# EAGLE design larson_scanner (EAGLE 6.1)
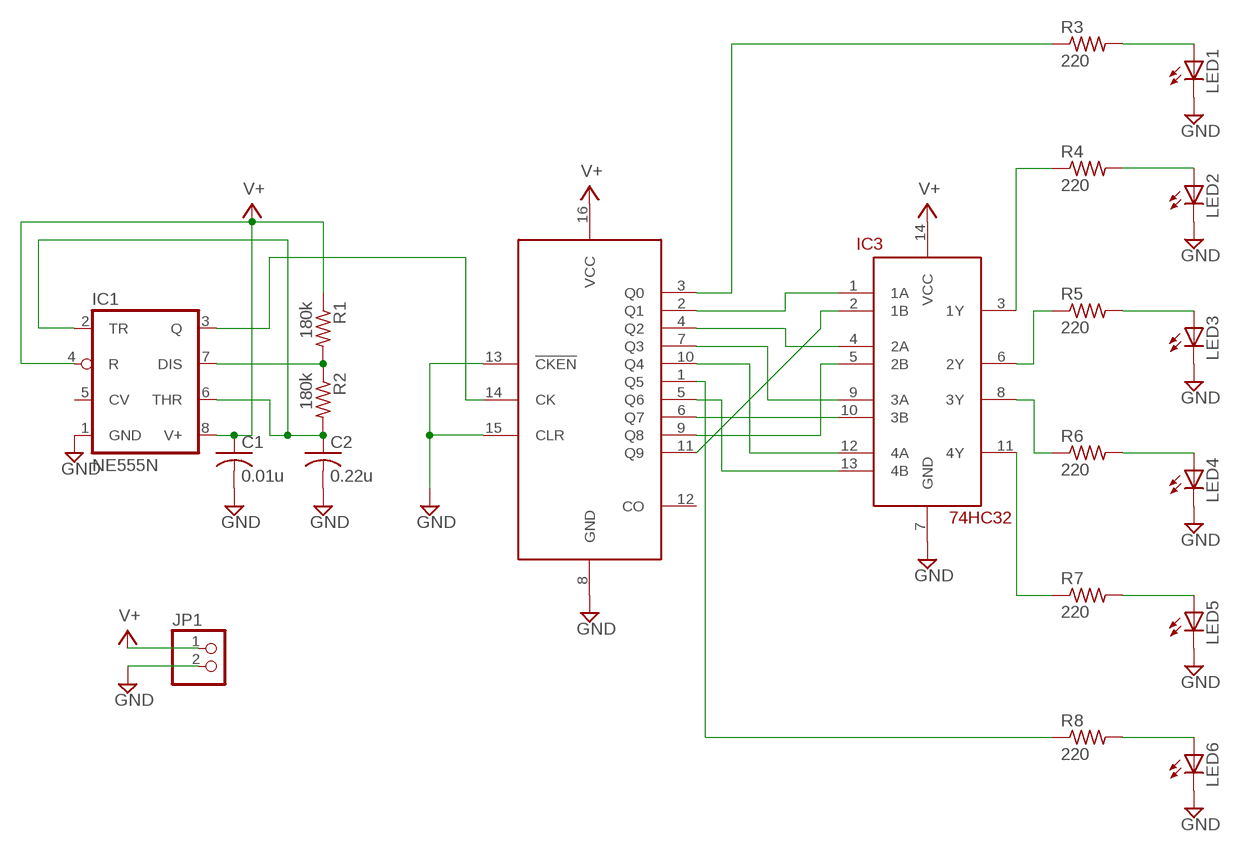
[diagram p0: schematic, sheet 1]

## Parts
C1  0.01u  C-US025-025X050  [C025-025X050]
C2  0.22u  C-US025-025X050  [C025-025X050]
IC1  NE555N  [DIL08]
IC2  74HC4017  [DIP16]
IC3  74HC32  [DIP14]
JP1  PINHD-1X2  [1X02]
LED1  LED5MM  [LED5MM]
LED2  LED5MM  [LED5MM]
LED3  LED5MM  [LED5MM]
LED4  LED5MM  [LED5MM]
LED5  LED5MM  [LED5MM]
LED6  LED5MM  [LED5MM]
R1  180k  R-US_0204/7  [0204/7]
R2  180k  R-US_0204/7  [0204/7]
R3  220  R-US_0204/7  [0204/7]
R4  220  R-US_0204/7  [0204/7]
R5  220  R-US_0204/7  [0204/7]
R6  220  R-US_0204/7  [0204/7]
R7  220  R-US_0204/7  [0204/7]
R8  220  R-US_0204/7  [0204/7]

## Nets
GND: C1.2 C2.2 IC1.1(GND) IC2.8(GND) IC2.13(!CKEN) IC2.15(CLR) IC3.7(GND) JP1.2 LED1.K(C) LED2.K(C) LED3.K(C) LED4.K(C) LED5.K(C) LED6.K(C)
N$1: LED4.A R6.2
N$2: LED3.A R5.2
N$3: LED2.A R4.2
N$4: LED1.A R3.2
N$5: LED5.A R7.2
N$6: LED6.A R8.2
N$7: IC2.1(Q5) R8.1
N$8: IC3.3(1Y) R4.1
N$9: IC3.6(2Y) R5.1
N$10: IC3.8(3Y) R6.1
N$11: IC2.3(Q0) R3.1
N$12: IC3.11(4Y) R7.1
N$13: IC2.2(Q1) IC3.1(1A)
N$14: IC2.4(Q2) IC3.4(2A)
N$15: IC2.7(Q3) IC3.9(3A)
N$16: IC2.10(Q4) IC3.12(4A)
N$17: IC2.5(Q6) IC3.13(4B)
N$18: IC2.6(Q7) IC3.10(3B)
N$19: IC2.9(Q8) IC3.5(2B)
N$20: IC2.11(Q9) IC3.2(1B)
N$21: IC1.7(DIS) R1.2 R2.1
N$22: C2.1 IC1.2(TR) IC1.6(THR) R2.2
N$23: IC1.3(Q) IC2.14(CK)
V+: C1.1 IC1.4(R) IC1.8(V+) IC2.16(VCC) IC3.14(VCC) JP1.1 R1.1
Unconnected: IC1.5(CV) IC2.12(CO)

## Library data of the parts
C1 C2 = rcl:C-US: CAPACITOR, American symbol
IC1 = linear:*555: TIMER
IC2 = jcm:74HC4017: Decimal counter with carry
IC3 = jcm:74HC32
JP1 = pinhead:PINHD-1X2: PIN HEADER
LED1-LED6 = led:LED: LED
R1-R8 = rcl:R-US_: RESISTOR, American symbol

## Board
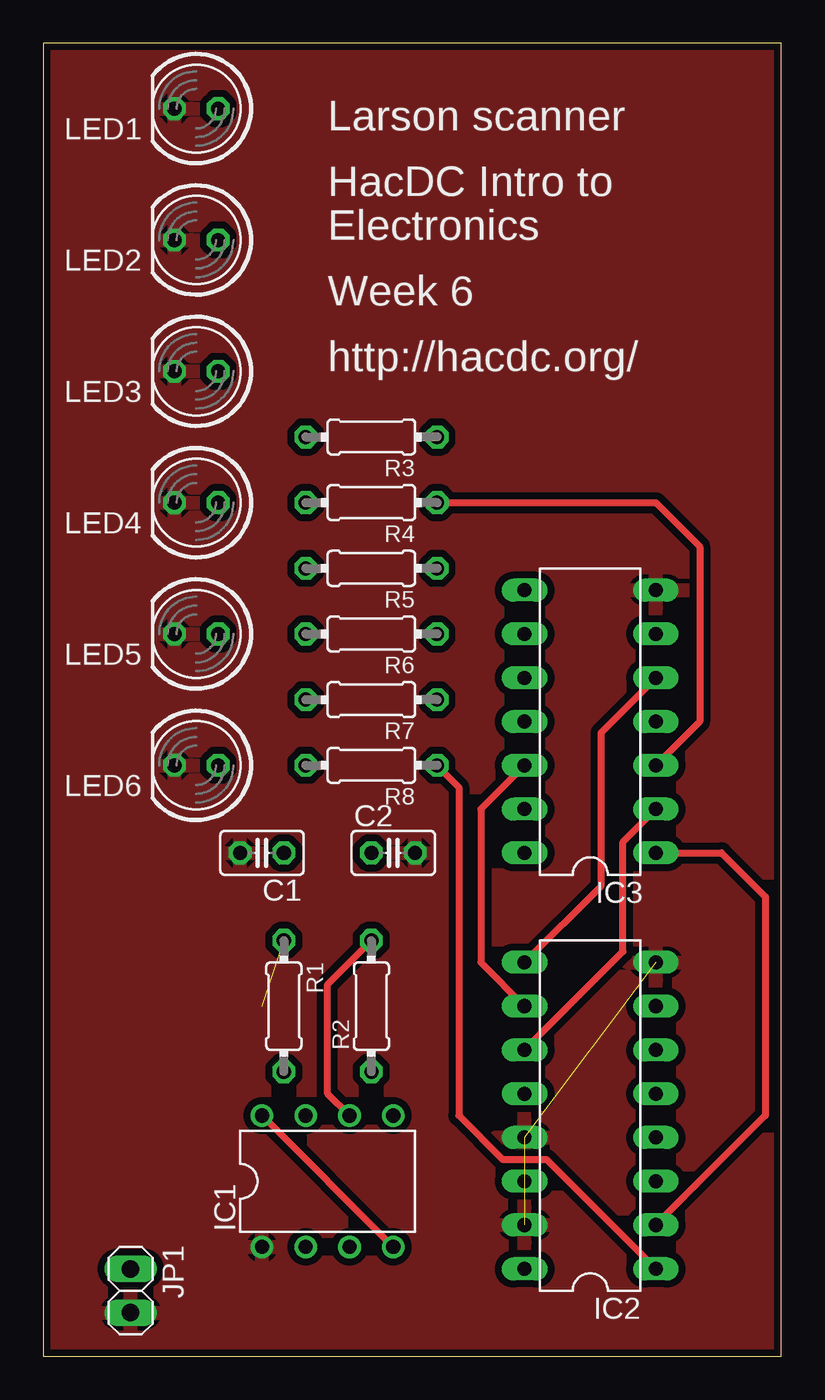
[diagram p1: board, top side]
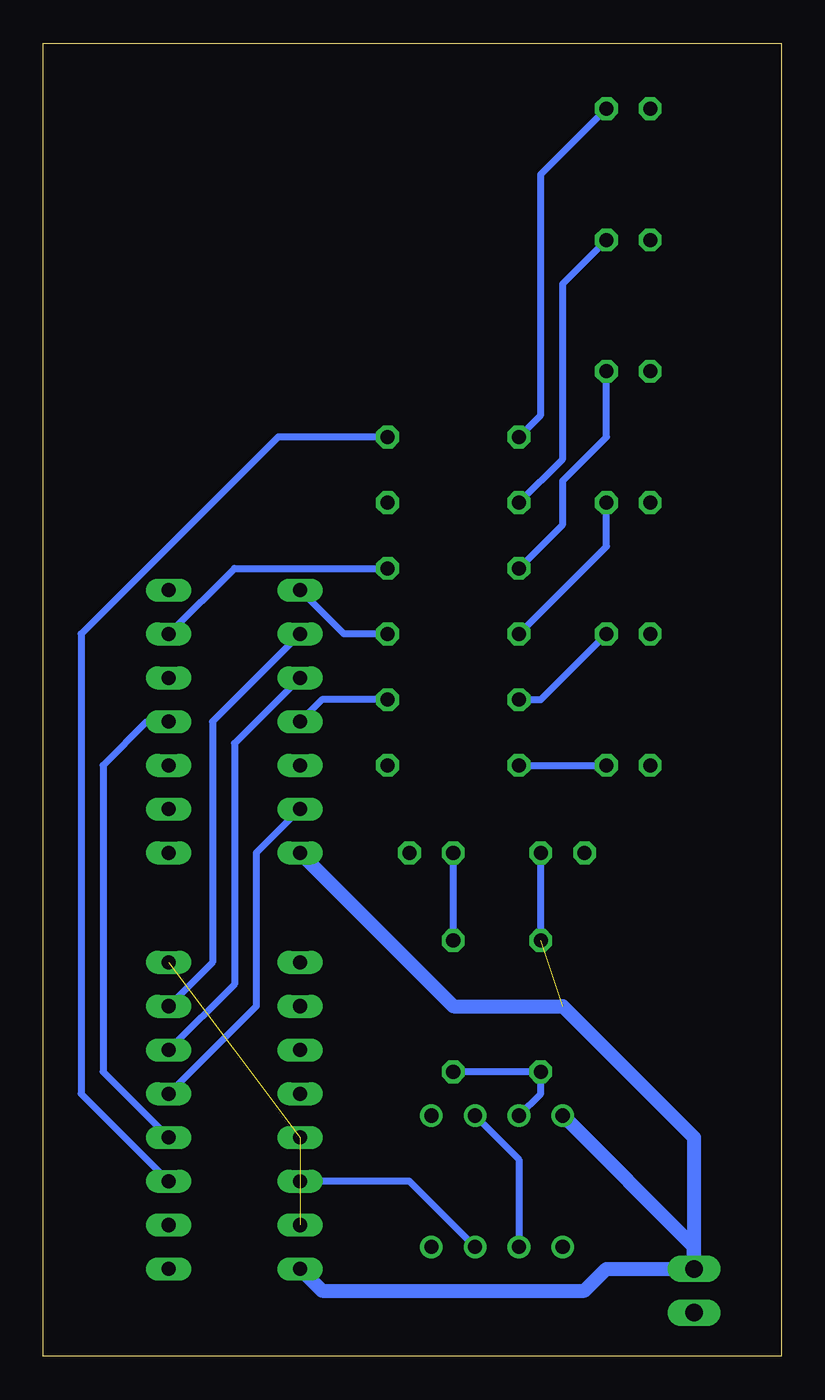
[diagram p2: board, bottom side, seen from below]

Size 42.85 x 76.19 mm. Coordinates in mm from the lower left corner, seen from the top.
Outline: 0,0 42.85,0 42.85,76.19 0,76.19 0,0
Copper layers (1*16): Top 0.035mm / dielectric 1.5mm / Bottom 0.035mm
Design rules: minimum track width 6mil, minimum drill 12mil, track to track 6mil, track to pad 6mil, pad to pad 6mil, via to via 6mil, smd to smd 0mil, copper to edge 10mil, drill to drill 10mil, minimum pad ring 10mil, minimum via ring 6mil, stop-mask expansion 2mil, vias tented up to drill 100mil, thermal gap 10mil

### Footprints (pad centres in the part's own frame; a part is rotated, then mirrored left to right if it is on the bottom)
C025-025X050 = drill 0.813 octagon: 1 -1.27,0; 2 1.27,0
DIL08 = drill 0.813 pad 1.27: 1 -3.81,-3.81; 2 -1.27,-3.81; 3 1.27,-3.81; 4 3.81,-3.81; 5 3.81,3.81; 6 1.27,3.81; 7 -1.27,3.81; 8 -3.81,3.81
DIP16 = drill 0.813 long: 1 -8.89,-3.81; 2 -6.35,-3.81; 3 -3.81,-3.81; 4 -1.27,-3.81; 5 1.27,-3.81; 6 3.81,-3.81; 7 6.35,-3.81; 8 8.89,-3.81; 9 8.89,3.81; 10 6.35,3.81; 11 3.81,3.81; 12 1.27,3.81; 13 -1.27,3.81; 14 -3.81,3.81; 15 -6.35,3.81; 16 -8.89,3.81
DIP14 = drill 0.813 long: 1 -7.62,-3.81; 2 -5.08,-3.81; 3 -2.54,-3.81; 4 0,-3.81; 5 2.54,-3.81; 6 5.08,-3.81; 7 7.62,-3.81; 8 7.62,3.81; 9 5.08,3.81; 10 2.54,3.81; 11 0,3.81; 12 -2.54,3.81; 13 -5.08,3.81; 14 -7.62,3.81
1X02 = drill 1.016 long: 1 -1.27,0; 2 1.27,0
LED5MM = drill 0.813 octagon: A -1.27,0; K 1.27,0
0204/7 = drill 0.813 octagon: 1 -3.81,0; 2 3.81,0

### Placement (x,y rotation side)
C1  12.7,29.21 180 top
C2  20.32,29.21 0 top
IC1  16.51,10.16 0 top
IC2  31.75,13.97 90 top
IC3  31.75,36.83 90 top
JP1  5.08,3.81 270 top
LED1  8.89,72.39 180 top
LED2  8.89,64.77 180 top
LED3  8.89,57.15 180 top
LED4  8.89,49.53 180 top
LED5  8.89,41.91 180 top
LED6  8.89,34.29 180 top
R1  13.97,20.32 270 top
R2  19.05,20.32 90 top
R3  19.05,53.34 180 top
R4  19.05,49.53 180 top
R5  19.05,45.72 180 top
R6  19.05,41.91 180 top
R7  19.05,38.1 180 top
R8  19.05,34.29 180 top

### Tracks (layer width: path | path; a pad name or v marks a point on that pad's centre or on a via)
GND  (2 unrouted)
  pour Top (isolate 0.406): -1.27,77.47 44.45,77.47 44.45,-1.27 -1.27,-1.27
N$1
  Bottom 0.406: R6.2 10.16,46.99 LED4.A
N$2
  Bottom 0.406: R5.2 12.7,48.26 12.7,50.8 10.16,53.34 LED3.A
N$3
  Bottom 0.406: R4.2 12.7,52.07 12.7,62.23 LED2.A
N$4
  Bottom 0.406: R3.2 13.97,54.61 13.97,68.58 LED1.A
N$5
  Bottom 0.406: R7.2 13.97,38.1 LED5.A
N$6
  Bottom 0.406: R8.2 LED6.A
N$7
  Top 0.406: R8.1 24.13,33.02 24.13,13.97 26.67,11.43 29.21,11.43 IC2.1
N$8
  Top 0.406: R4.1 35.56,49.53 38.1,46.99 38.1,36.83 IC3.3
N$9
  Bottom 0.406: IC3.6 31.75,45.72 R5.1
N$10
  Bottom 0.406: R6.1 25.4,41.91 IC3.8
N$11
  Bottom 0.406: R3.1 29.21,53.34 40.64,41.91 40.64,15.24 IC2.3
N$12
  Bottom 0.406: R7.1 26.67,38.1 IC3.11
N$13
  Top 0.406: IC3.1 39.37,29.21 41.91,26.67 41.91,13.97 IC2.2
N$14
  Bottom 0.406: IC3.4 36.83,36.83 39.37,34.29 39.37,16.51 IC2.4
N$15
  Bottom 0.406: IC3.9 33.02,36.83 33.02,22.86 IC2.7
N$16
  Top 0.406: IC3.12 25.4,31.75 25.4,22.86 IC2.10
N$17
  Bottom 0.406: IC3.13 30.48,29.21 30.48,20.32 IC2.5
N$18
  Bottom 0.406: IC3.10 31.75,35.56 31.75,21.59 IC2.6
N$19
  Top 0.406: IC2.9 32.38,27.3 32.38,36.2 IC3.5
N$20
  Top 0.406: IC2.11 33.66,23.5 33.66,29.84 IC3.2
N$21
  Bottom 0.406: R2.1 R1.2 13.97,15.24 IC1.7
N$22
  Top 0.406: IC1.6 16.51,15.24 16.51,21.59 R2.2
  Bottom 0.406: R2.2 C2.1 | IC1.6 15.24,11.43 IC1.2
N$23
  Bottom 0.406: IC1.3 21.59,10.16 IC2.14
V+  (1 unrouted)
  Top 0.406: IC1.8 IC1.4
  Bottom 0.406: R1.1 C1.1
  Bottom 0.813: JP1.1 5.08,6.35 IC1.8 | IC2.16 26.67,3.81 11.43,3.81 10.16,5.08 JP1.1 | IC3.14 19.05,20.32 12.7,20.32 5.08,12.7 JP1.1

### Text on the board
tNames: Larson scanner | HacDC Intro to | Electronics | Week 6 | http://hacdc.org/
